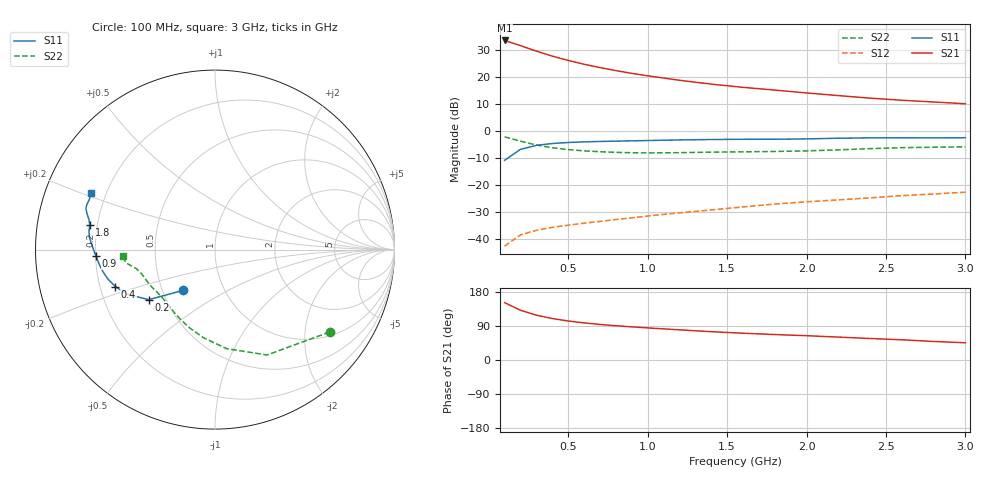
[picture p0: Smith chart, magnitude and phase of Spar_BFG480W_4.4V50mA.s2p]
! Filename: 4_450BFG480.001
! Title: BFG480W
! Bias: Vce=4.4V; Ic=50mA
! Company: NXP Semiconductors NL
! User: Quality&Reliability T&D
! Measure time: 10 Nov 1999 / 12:06:01
#  MHz  S  MA  R 50
! Freq  S11  S21  S12  S22  :
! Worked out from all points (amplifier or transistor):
!   20 points, 100 MHz to 3 GHz, reference 50 ohm
!   highest |S21| = 33.6 dB at 100 MHz (marker M1)
!   |S21| within 3 dB of that: start of sweep to 253.3 MHz
!   unconditionally stable (mu >= 1): 950 MHz to end of sweep
!   at 400 MHz: K = 0.65, MSG = 31.7 dB, |S12| = -35.6 dB
!   at 1.2 GHz: K = 1.05, MAG = 23.1 dB, |S12| = -30.2 dB
!   at 3 GHz: K = 1.06, MAG = 14.9 dB, |S12| = -22.6 dB
!   S11 on the Smith chart (normalised r, x): 100 MHz: 0.64, -0.32; 200 MHz: 0.40, -0.29; 400 MHz: 0.26, -0.17; 900 MHz: 0.20, -0.03; 1.8 GHz: 0.17, +0.09; 3 GHz: 0.14, +0.21
100  0.2895 -128.2  47.9 151.3  0.007454 64.0  0.7862 -35.8
200  0.4624 -142.9  38.43 131.2  0.01207 55.7  0.6547 -63.8
300  0.548 -153.0  30.39 118.3  0.01469 52.3  0.5552 -83.4
400  0.5927 -159.7  24.57 109.4  0.01664 52.1  0.4942 -97.7
500  0.6191 -164.7  20.45 103.0  0.01825 53.4  0.4571 -108.4
600  0.6354 -168.6  17.38 97.9  0.01985 54.9  0.4333 -116.5
700  0.6466 -171.7  15.08 93.9  0.02144 57.0  0.4173 -123.0
800  0.6555 -174.4  13.26 90.4  0.02319 59.1  0.4066 -128.4
900  0.6641 -176.9  11.79 87.5  0.02494 61.4  0.4001 -133.1
1000  0.673 -179.1  10.62 84.7  0.02697 63.0  0.3973 -137.4
1200  0.6899 177.2  8.784 79.6  0.03087 65.8  0.4011 -144.4
1400  0.7028 174.5  7.45 74.7  0.03489 67.9  0.4098 -149.6
1600  0.7095 171.8  6.499 70.7  0.03969 69.7  0.4158 -153.6
1800  0.7108 169.0  5.779 67.2  0.04489 71.1  0.4224 -157.7
2000  0.7217 166.6  5.114 64.1  0.04945 72.5  0.4326 -162.4
2200  0.7418 164.2  4.568 60.5  0.05367 72.9  0.4516 -166.5
2400  0.7549 162.3  4.098 56.7  0.05838 73.0  0.4763 -169.2
2600  0.7569 160.6  3.747 53.3  0.06428 72.7  0.4961 -171.0
2800  0.7537 158.3  3.477 48.9  0.06899 71.7  0.5059 -172.9
3000  0.7589 155.6  3.228 45.4  0.07429 71.2  0.5135 -176.0
